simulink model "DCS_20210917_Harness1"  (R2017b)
settings: Solver=FixedStepDiscrete  StartTime=0.0  StopTime=10.0  FixedStep=0.01  RelTol=1e-3  EnableMultiTasking=on
undefined symbols (not defined in the file): sigbuilder_block
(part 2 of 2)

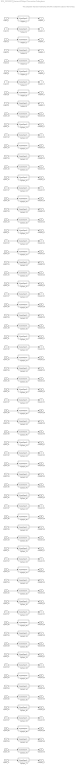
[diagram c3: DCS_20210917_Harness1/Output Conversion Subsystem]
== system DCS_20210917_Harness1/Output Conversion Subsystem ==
  note: This subsystem has been inserted by Simulink to adapt the output of the harnessed component to the interface required by the sink blocks. Modifying the contents of this subsystem may result in compilation and simulation failure.
  Inport_1 : Inport
  Inport_2 : Inport  Port=2
  Inport_3 : Inport  Port=3
  Inport_4 : Inport  Port=4
  Inport_5 : Inport  Port=5
  Inport_6 : Inport  Port=6
  Inport_7 : Inport  Port=7
  Inport_8 : Inport  Port=8
  Inport_9 : Inport  Port=9
  Inport_10 : Inport  Port=10
  Inport_11 : Inport  Port=11
  Inport_12 : Inport  Port=12
  Inport_13 : Inport  Port=13
  Inport_14 : Inport  Port=14
  Inport_15 : Inport  Port=15
  Inport_16 : Inport  Port=16
  Inport_17 : Inport  Port=17
  Inport_18 : Inport  Port=18
  Inport_19 : Inport  Port=19
  Inport_20 : Inport  Port=20
  Inport_21 : Inport  Port=21
  Inport_22 : Inport  Port=22
  Inport_23 : Inport  Port=23
  Inport_24 : Inport  Port=24
  Inport_25 : Inport  Port=25
  Inport_26 : Inport  Port=26
  Inport_27 : Inport  Port=27
  Inport_28 : Inport  Port=28
  Inport_29 : Inport  Port=29
  Inport_30 : Inport  Port=30
  Inport_31 : Inport  Port=31
  Inport_32 : Inport  Port=32
  Inport_33 : Inport  Port=33
  Inport_34 : Inport  Port=34
  Inport_35 : Inport  Port=35
  Inport_36 : Inport  Port=36
  Inport_37 : Inport  Port=37
  Inport_38 : Inport  Port=38
  Inport_39 : Inport  Port=39
  Inport_40 : Inport  Port=40
  Inport_41 : Inport  Port=41
  Inport_42 : Inport  Port=42
  Inport_43 : Inport  Port=43
  Inport_44 : Inport  Port=44
  Inport_45 : Inport  Port=45
  Inport_46 : Inport  Port=46
  Inport_47 : Inport  Port=47
  Inport_48 : Inport  Port=48
  Inport_49 : Inport  Port=49
  Inport_50 : Inport  Port=50
  Inport_51 : Inport  Port=51
  Inport_52 : Inport  Port=52
  Inport_53 : Inport  Port=53
  Inport_54 : Inport  Port=54
  Inport_55 : Inport  Port=55
  Inport_56 : Inport  Port=56
  Inport_57 : Inport  Port=57
  Inport_58 : Inport  Port=58
  Inport_59 : Inport  Port=59
  Inport_60 : Inport  Port=60
  Inport_61 : Inport  Port=61
  Inport_62 : Inport  Port=62
  Inport_63 : Inport  Port=63
  Inport_64 : Inport  Port=64
  Inport_65 : Inport  Port=65
  Inport_66 : Inport  Port=66
  Inport_67 : Inport  Port=67
  Inport_68 : Inport  Port=68
  Inport_69 : Inport  Port=69
  Inport_70 : Inport  Port=70
  Inport_71 : Inport  Port=71
  SigSpec_{1,5,19,22,24,27} (6 alike) : SignalSpecification  OutDataTypeStr=fixdt('ufix16_Sp1')  Unit=V  Dimensions=[1]  SampleTime=0.01
  SigSpec_10 : SignalSpecification  OutDataTypeStr=fixdt('ufix8_B1985')  Unit=Y  Dimensions=[1]  SampleTime=0.01
  SigSpec_11 : SignalSpecification  OutDataTypeStr=uint32  Unit=numb  Dimensions=[1]  SampleTime=0.01
  SigSpec_{3,12,26,38..58,64..70} (31 alike) : SignalSpecification  OutDataTypeStr=uint8  Unit=enum  Dimensions=[1]  SampleTime=0.01
  SigSpec_{13,23,30,71} (4 alike) : SignalSpecification  OutDataTypeStr=uint8  Unit=numb  Dimensions=[1]  SampleTime=0.01
  SigSpec_14 : SignalSpecification  OutDataTypeStr=uint8  Unit=numb  Dimensions=[17]  SampleTime=0.01
  SigSpec_15 : SignalSpecification  OutDataTypeStr=uint8  Unit=numb  Dimensions=[8]  SampleTime=0.01
  SigSpec_16 : SignalSpecification  OutDataTypeStr=single  Unit=V  Dimensions=[1]  SampleTime=0.01
  SigSpec_17 : SignalSpecification  OutDataTypeStr=fixdt('ufix16_Sp1_Bn400')  Unit=A  Dimensions=[1]  SampleTime=0.01
  SigSpec_18 : SignalSpecification  OutDataTypeStr=fixdt('ufix16_Sp1')  Unit=kWh  Dimensions=[1]  SampleTime=0.01
  SigSpec_2 : SignalSpecification  OutDataTypeStr=uint32  Unit=numb  Dimensions=[1]  SampleTime=0.01
  SigSpec_{20,34,36,62..63} (5 alike) : SignalSpecification  OutDataTypeStr=fixdt('ufix8_Bn50')  Unit=C  Dimensions=[1]  SampleTime=0.01
  SigSpec_21 : SignalSpecification  OutDataTypeStr=fixdt('ufix16_Sp1')  Unit=%  Dimensions=[1]  SampleTime=0.01
  SigSpec_25 : SignalSpecification  OutDataTypeStr=fixdt('ufix16_Sp1_Bn400')  Unit=A  Dimensions=[1]  SampleTime=0.01
  SigSpec_28 : SignalSpecification  OutDataTypeStr=fixdt('ufix16_Sp1_Bn400')  Unit=A  Dimensions=[1]  SampleTime=0.01
  SigSpec_29 : SignalSpecification  OutDataTypeStr=fixdt('ufix16_Sp01')  Unit=V  Dimensions=[1]  SampleTime=0.01
  SigSpec_31 : SignalSpecification  OutDataTypeStr=uint8  Unit=pct  Dimensions=[1]  SampleTime=0.01
  SigSpec_32 : SignalSpecification  OutDataTypeStr=uint16  Unit=Min  Dimensions=[1]  SampleTime=0.01
  SigSpec_33 : SignalSpecification  OutDataTypeStr=fixdt('ufix8_B1')  Unit=numb  Dimensions=[1]  SampleTime=0.01
  SigSpec_35 : SignalSpecification  OutDataTypeStr=fixdt('ufix8_B1')  Unit=numb  Dimensions=[1]  SampleTime=0.01
  SigSpec_37 : SignalSpecification  OutDataTypeStr=fixdt('ufix8_B1')  Unit=numb  Dimensions=[1]  SampleTime=0.01
  SigSpec_4 : SignalSpecification  OutDataTypeStr=fixdt('ufix16_Sp1')  Unit=Ah  Dimensions=[1]  SampleTime=0.01
  SigSpec_59 : SignalSpecification  OutDataTypeStr=uint8  Unit=%  Dimensions=[1]  SampleTime=0.01
  SigSpec_6 : SignalSpecification  OutDataTypeStr=uint8  Unit=numb  Dimensions=[4]  SampleTime=0.01
  SigSpec_60 : SignalSpecification  OutDataTypeStr=fixdt('ufix16_Sp01')  Unit=V  Dimensions=[1]  SampleTime=0.01
  SigSpec_61 : SignalSpecification  OutDataTypeStr=fixdt('ufix16_Sp01')  Unit=V  Dimensions=[1]  SampleTime=0.01
  SigSpec_7 : SignalSpecification  OutDataTypeStr=uint32  Unit=numb  Dimensions=[1]  SampleTime=0.01
  SigSpec_8 : SignalSpecification  OutDataTypeStr=uint8  Unit=D  Dimensions=[1]  SampleTime=0.01
  SigSpec_9 : SignalSpecification  OutDataTypeStr=uint8  Unit=M  Dimensions=[1]  SampleTime=0.01
  Outport_1 : Outport
  Outport_2 : Outport  Port=2
  Outport_3 : Outport  Port=3
  Outport_4 : Outport  Port=4
  Outport_5 : Outport  Port=5
  Outport_6 : Outport  Port=6
  Outport_7 : Outport  Port=7
  Outport_8 : Outport  Port=8
  Outport_9 : Outport  Port=9
  Outport_10 : Outport  Port=10
  Outport_11 : Outport  Port=11
  Outport_12 : Outport  Port=12
  Outport_13 : Outport  Port=13
  Outport_14 : Outport  Port=14
  Outport_15 : Outport  Port=15
  Outport_16 : Outport  Port=16
  Outport_17 : Outport  Port=17
  Outport_18 : Outport  Port=18
  Outport_19 : Outport  Port=19
  Outport_20 : Outport  Port=20
  Outport_21 : Outport  Port=21
  Outport_22 : Outport  Port=22
  Outport_23 : Outport  Port=23
  Outport_24 : Outport  Port=24
  Outport_25 : Outport  Port=25
  Outport_26 : Outport  Port=26
  Outport_27 : Outport  Port=27
  Outport_28 : Outport  Port=28
  Outport_29 : Outport  Port=29
  Outport_30 : Outport  Port=30
  Outport_31 : Outport  Port=31
  Outport_32 : Outport  Port=32
  Outport_33 : Outport  Port=33
  Outport_34 : Outport  Port=34
  Outport_35 : Outport  Port=35
  Outport_36 : Outport  Port=36
  Outport_37 : Outport  Port=37
  Outport_38 : Outport  Port=38
  Outport_39 : Outport  Port=39
  Outport_40 : Outport  Port=40
  Outport_41 : Outport  Port=41
  Outport_42 : Outport  Port=42
  Outport_43 : Outport  Port=43
  Outport_44 : Outport  Port=44
  Outport_45 : Outport  Port=45
  Outport_46 : Outport  Port=46
  Outport_47 : Outport  Port=47
  Outport_48 : Outport  Port=48
  Outport_49 : Outport  Port=49
  Outport_50 : Outport  Port=50
  Outport_51 : Outport  Port=51
  Outport_52 : Outport  Port=52
  Outport_53 : Outport  Port=53
  Outport_54 : Outport  Port=54
  Outport_55 : Outport  Port=55
  Outport_56 : Outport  Port=56
  Outport_57 : Outport  Port=57
  Outport_58 : Outport  Port=58
  Outport_59 : Outport  Port=59
  Outport_60 : Outport  Port=60
  Outport_61 : Outport  Port=61
  Outport_62 : Outport  Port=62
  Outport_63 : Outport  Port=63
  Outport_64 : Outport  Port=64
  Outport_65 : Outport  Port=65
  Outport_66 : Outport  Port=66
  Outport_67 : Outport  Port=67
  Outport_68 : Outport  Port=68
  Outport_69 : Outport  Port=69
  Outport_70 : Outport  Port=70
  Outport_71 : Outport  Port=71
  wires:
  Inport_1/1 -> SigSpec_1/1
  SigSpec_1/1 -> Outport_1/1
  Inport_2/1 -> SigSpec_2/1
  SigSpec_2/1 -> Outport_2/1
  Inport_3/1 -> SigSpec_3/1
  SigSpec_3/1 -> Outport_3/1
  Inport_4/1 -> SigSpec_4/1
  SigSpec_4/1 -> Outport_4/1
  Inport_5/1 -> SigSpec_5/1
  SigSpec_5/1 -> Outport_5/1
  Inport_6/1 -> SigSpec_6/1
  SigSpec_6/1 -> Outport_6/1
  Inport_7/1 -> SigSpec_7/1
  SigSpec_7/1 -> Outport_7/1
  Inport_8/1 -> SigSpec_8/1
  SigSpec_8/1 -> Outport_8/1
  Inport_9/1 -> SigSpec_9/1
  SigSpec_9/1 -> Outport_9/1
  Inport_10/1 -> SigSpec_10/1
  SigSpec_10/1 -> Outport_10/1
  Inport_11/1 -> SigSpec_11/1
  SigSpec_11/1 -> Outport_11/1
  Inport_12/1 -> SigSpec_12/1
  SigSpec_12/1 -> Outport_12/1
  Inport_13/1 -> SigSpec_13/1
  SigSpec_13/1 -> Outport_13/1
  Inport_14/1 -> SigSpec_14/1
  SigSpec_14/1 -> Outport_14/1
  Inport_15/1 -> SigSpec_15/1
  SigSpec_15/1 -> Outport_15/1
  Inport_16/1 -> SigSpec_16/1
  SigSpec_16/1 -> Outport_16/1
  Inport_17/1 -> SigSpec_17/1
  SigSpec_17/1 -> Outport_17/1
  Inport_18/1 -> SigSpec_18/1
  SigSpec_18/1 -> Outport_18/1
  Inport_19/1 -> SigSpec_19/1
  SigSpec_19/1 -> Outport_19/1
  Inport_20/1 -> SigSpec_20/1
  SigSpec_20/1 -> Outport_20/1
  Inport_21/1 -> SigSpec_21/1
  SigSpec_21/1 -> Outport_21/1
  Inport_22/1 -> SigSpec_22/1
  SigSpec_22/1 -> Outport_22/1
  Inport_23/1 -> SigSpec_23/1
  SigSpec_23/1 -> Outport_23/1
  Inport_24/1 -> SigSpec_24/1
  SigSpec_24/1 -> Outport_24/1
  Inport_25/1 -> SigSpec_25/1
  SigSpec_25/1 -> Outport_25/1
  Inport_26/1 -> SigSpec_26/1
  SigSpec_26/1 -> Outport_26/1
  Inport_27/1 -> SigSpec_27/1
  SigSpec_27/1 -> Outport_27/1
  Inport_28/1 -> SigSpec_28/1
  SigSpec_28/1 -> Outport_28/1
  Inport_29/1 -> SigSpec_29/1
  SigSpec_29/1 -> Outport_29/1
  Inport_30/1 -> SigSpec_30/1
  SigSpec_30/1 -> Outport_30/1
  Inport_31/1 -> SigSpec_31/1
  SigSpec_31/1 -> Outport_31/1
  Inport_32/1 -> SigSpec_32/1
  SigSpec_32/1 -> Outport_32/1
  Inport_33/1 -> SigSpec_33/1
  SigSpec_33/1 -> Outport_33/1
  Inport_34/1 -> SigSpec_34/1
  SigSpec_34/1 -> Outport_34/1
  Inport_35/1 -> SigSpec_35/1
  SigSpec_35/1 -> Outport_35/1
  Inport_36/1 -> SigSpec_36/1
  SigSpec_36/1 -> Outport_36/1
  Inport_37/1 -> SigSpec_37/1
  SigSpec_37/1 -> Outport_37/1
  Inport_38/1 -> SigSpec_38/1
  SigSpec_38/1 -> Outport_38/1
  Inport_39/1 -> SigSpec_39/1
  SigSpec_39/1 -> Outport_39/1
  Inport_40/1 -> SigSpec_40/1
  SigSpec_40/1 -> Outport_40/1
  Inport_41/1 -> SigSpec_41/1
  SigSpec_41/1 -> Outport_41/1
  Inport_42/1 -> SigSpec_42/1
  SigSpec_42/1 -> Outport_42/1
  Inport_43/1 -> SigSpec_43/1
  SigSpec_43/1 -> Outport_43/1
  Inport_44/1 -> SigSpec_44/1
  SigSpec_44/1 -> Outport_44/1
  Inport_45/1 -> SigSpec_45/1
  SigSpec_45/1 -> Outport_45/1
  Inport_46/1 -> SigSpec_46/1
  SigSpec_46/1 -> Outport_46/1
  Inport_47/1 -> SigSpec_47/1
  SigSpec_47/1 -> Outport_47/1
  Inport_48/1 -> SigSpec_48/1
  SigSpec_48/1 -> Outport_48/1
  Inport_49/1 -> SigSpec_49/1
  SigSpec_49/1 -> Outport_49/1
  Inport_50/1 -> SigSpec_50/1
  SigSpec_50/1 -> Outport_50/1
  Inport_51/1 -> SigSpec_51/1
  SigSpec_51/1 -> Outport_51/1
  Inport_52/1 -> SigSpec_52/1
  SigSpec_52/1 -> Outport_52/1
  Inport_53/1 -> SigSpec_53/1
  SigSpec_53/1 -> Outport_53/1
  Inport_54/1 -> SigSpec_54/1
  SigSpec_54/1 -> Outport_54/1
  Inport_55/1 -> SigSpec_55/1
  SigSpec_55/1 -> Outport_55/1
  Inport_56/1 -> SigSpec_56/1
  SigSpec_56/1 -> Outport_56/1
  Inport_57/1 -> SigSpec_57/1
  SigSpec_57/1 -> Outport_57/1
  Inport_58/1 -> SigSpec_58/1
  SigSpec_58/1 -> Outport_58/1
  Inport_59/1 -> SigSpec_59/1
  SigSpec_59/1 -> Outport_59/1
  Inport_60/1 -> SigSpec_60/1
  SigSpec_60/1 -> Outport_60/1
  Inport_61/1 -> SigSpec_61/1
  SigSpec_61/1 -> Outport_61/1
  Inport_62/1 -> SigSpec_62/1
  SigSpec_62/1 -> Outport_62/1
  Inport_63/1 -> SigSpec_63/1
  SigSpec_63/1 -> Outport_63/1
  Inport_64/1 -> SigSpec_64/1
  SigSpec_64/1 -> Outport_64/1
  Inport_65/1 -> SigSpec_65/1
  SigSpec_65/1 -> Outport_65/1
  Inport_66/1 -> SigSpec_66/1
  SigSpec_66/1 -> Outport_66/1
  Inport_67/1 -> SigSpec_67/1
  SigSpec_67/1 -> Outport_67/1
  Inport_68/1 -> SigSpec_68/1
  SigSpec_68/1 -> Outport_68/1
  Inport_69/1 -> SigSpec_69/1
  SigSpec_69/1 -> Outport_69/1
  Inport_70/1 -> SigSpec_70/1
  SigSpec_70/1 -> Outport_70/1
  Inport_71/1 -> SigSpec_71/1
  SigSpec_71/1 -> Outport_71/1
